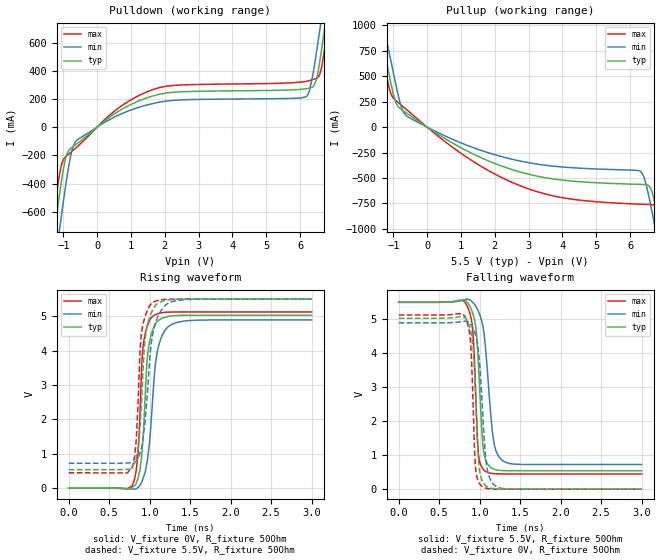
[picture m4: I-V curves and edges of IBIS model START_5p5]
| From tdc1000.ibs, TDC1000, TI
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|   Model
[Model]   START_5p5
Model_type   Output
Polarity   Non-Inverting
Vmeas = 2.25
Vref = 0
Cref = 1pF
Rref = 100000
|   typ   min   max
C_comp   3.839pF   2.875pF   5.918pF
[Voltage Range]   5.5   5.499   5.501
[Temperature Range]   27   125   -40
[Pullup Reference]   5.5   5.499   5.501
[Pulldown Reference]   0   0   0
[Power Clamp Reference]   5.5   5.499   5.501
[GND Clamp Reference]   0   0   0
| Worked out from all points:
|   slope of the pulldown table from 0 to 0.825 V, typ, clamps not added: 5.93 ohm
|   slope of the pullup table from 0 to 0.825 V, typ, clamps not added: 4.85 ohm
|   falling waveform, V_fixture 5.5V, R_fixture 50Ohm: 20-80 % time 70ps typ, 102ps min, 53ps max; typ from 5.5 V to 0.54 V
|   rising waveform, V_fixture 0V, R_fixture 50Ohm: 20-80 % time 78.9ps typ, 110ps min, 62.3ps max; typ from 0 V to 5.03 V
|   rising waveform, V_fixture 5.5V, R_fixture 50Ohm: 20-80 % time 81.2ps typ, 114ps min, 63.2ps max; typ from 0.54 V to 5.5 V
|   falling waveform, V_fixture 0V, R_fixture 50Ohm: 20-80 % time 58ps typ, 81.7ps min, 46.1ps max; typ from 5.03 V to 0 V
[Pulldown]
|   Voltage   I(typ)   I(min)   I(max)
-5.5V     -8.662A    -8.76A     -8.611A
-1.359V   -923.6mA   -1.178A    -761.4mA
-1.111V   -477.3mA   -727.4mA   -335.6mA
-913mV    -204.1mA   -388.1mA   -205.8mA
-682mV    -132.8mA   -121.5mA   -158.6mA
522.5mV   96.45mA    72.9mA     115.7mA
2.024V    241.6mA    184.1mA    289.4mA
6.165V    271.7mA    214.3mA    324.2mA
6.479V    333.5mA    522.2mA    346.6mA
6.628V    536mA      758.7mA    413.8mA
6.875V    950.4mA    1.154A     810.8mA
11V       7.935A     7.845A     8.023A
[Pullup]
|   Voltage   I(typ)   I(min)   I(max)
-5.5V     7.938A     7.849A     8.028A
-2.926V   3.563A     3.648A     3.517A
-1.375V   940.5mA    1.139A     806.4mA
-1.078V   442.5mA    663.7mA    335.4mA
-896.5mV  220.7mA    374.8mA    253.5mA
-616mV    140.1mA    113mA      174.6mA
3.014V    -464.1mA   -350.5mA   -609.1mA
6.298V    -563mA     -432.3mA   -758mA
6.611V    -602.6mA   -770.2mA   -762.6mA
6.793V    -844.9mA   -1.087A    -788.1mA
7.024V    -1.258A    -1.508A    -1.108A
11V       -8.686A    -8.785A    -8.635A
[Ramp]
R_load = 50
|   typ   min   max
dV/dt_r   3.01915/7.8876e-11   2.93678/1.09594e-10   3.07578/6.23079e-11
dV/dt_f   2.97592/6.99651e-11   2.86404/1.01698e-10   3.03261/5.29874e-11
[Falling Waveform]
V_fixture = 5.5V
V_fixture_min = 5.499V
V_fixture_max = 5.501V
R_fixture = 50Ohm
C_fixture = 0F
|   Time   V(typ)   V(min)   V(max)
0s        5.5V       5.499V     5.501V
833ps     5.535V     5.591V     5.443V
916.4ps   5.162V     5.492V     4.651V
956.2ps   4.697V     5.365V     2.476V
991.5ps   3.382V     5.194V     906.3mV
1.043ns   1.222V     4.759V     590.4mV
1.078ns   839.1mV    4.008V     515.2mV
1.178ns   588.6mV    1.342V     456.4mV
1.276ns   548mV      852.2mV    448.1mV
3ns       540.1mV    725.6mV    446.6mV
[Rising Waveform]
V_fixture = 0V
V_fixture_min = 0V
V_fixture_max = 0V
R_fixture = 50Ohm
C_fixture = 0F
|   Time   V(typ)   V(min)   V(max)
0s        556.2nV    32.21uV    18.71uV
785.6ps   18.59mV    -23.16mV   72.17mV
854.6ps   273.4mV    18.34mV    952.4mV
908.6ps   1.142V     212.6mV    3.845V
927.2ps   1.803V     343.5mV    4.261V
977.6ps   3.927V     911.3mV    4.761V
1.052ns   4.683V     3.088V     5.022V
1.134ns   4.917V     4.323V     5.096V
1.315ns   5.019V     4.804V     5.125V
3ns       5.032V     4.895V     5.126V
[Rising Waveform]
V_fixture = 5.5V
V_fixture_min = 5.499V
V_fixture_max = 5.501V
R_fixture = 50Ohm
C_fixture = 0F
|   Time   V(typ)   V(min)   V(max)
0s        540.1mV    725.7mV    446.6mV
785.6ps   630.7mV    745.3mV    601.9mV
833ps     859.7mV    789.4mV    1.36V
880ps     1.729V     1.019V     3.935V
898.6ps   2.482V     1.174V     4.496V
945.1ps   4.352V     1.965V     5.005V
1.032ns   5.156V     4.393V     5.392V
1.117ns   5.404V     5.067V     5.469V
1.276ns   5.485V     5.427V     5.498V
3ns       5.5V       5.499V     5.501V
[Falling Waveform]
|Gnd
V_fixture = 0V
V_fixture_min = 0V
V_fixture_max = 0V
R_fixture = 50Ohm
C_fixture = 0F
|   Time   V(typ)   V(min)   V(max)
0s        5.032V     4.895V     5.126V
814.5ps   5.045V     4.943V     5.098V
880ps     4.752V     4.886V     4.528V
920.9ps   4.136V     4.718V     2.355V
952.9ps   2.599V     4.5V       538.9mV
988.5ps   749.7mV    3.959V     206mV
1.032ns   253.8mV    2.496V     76.79mV
1.084ns   88.68mV    718mV      25.3mV
1.2ns     8.766mV    87.48mV    2.373mV
3ns       3.548uV    25.94uV    18.77uV
